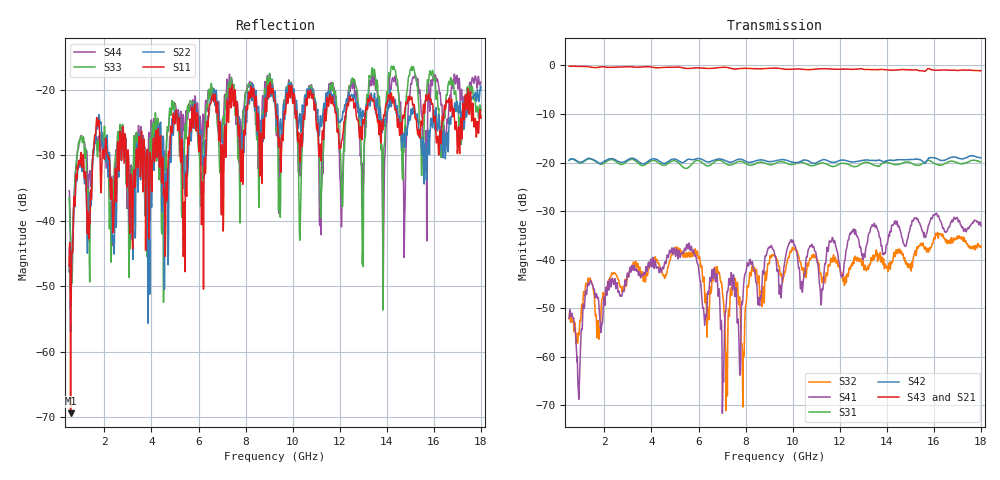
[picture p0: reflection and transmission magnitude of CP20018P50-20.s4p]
! Amtery
! Email: info@amtery.com
! Phone: 886-2-7730-0804
! Model Number: CP20018P-20
! 4-port S-parameter measurement data for Bi-Directional Coupler
! Frequency Range: 0.5 GHz to 18 GHz
! Port 1: Input
! Port 2: Output
! Port 3: Coupled Forward
! Port 4: Coupled Reverse
# hz S ma R 50
! freq  magS11  angS11  magS12  angS12  magS13  angS13  magS14  angS14
!  magS21  angS21  magS22  angS22  magS23  angS23  magS24  angS24
!  magS31  angS31  magS32  angS32  magS33  angS33  magS34  angS34
!  magS41  angS41  magS42  angS42  magS43  angS43  magS44  angS44
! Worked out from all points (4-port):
!   1401 points, 500 MHz to 18 GHz, reference 50 ohm
!   strongest paths, dB at 500 MHz, 4.875 GHz, 9.25 GHz, 13.62 GHz, 18 GHz:
!     S43: -0.1, -0.4, -0.5, -0.9, -1.1
!     S21: -0.1, -0.4, -0.7, -0.7, -1.0
!     S42: -19.5, -19.3, -19.7, -19.5, -19.0
!     S31: -19.5, -19.7, -20.2, -20.7, -19.8
!     S41: -52.1, -37.5, -39.4, -34.0, -33.0
!     S32: -52.1, -39.0, -39.2, -39.1, -37.1
!   lowest |S11| = -69.4 dB at 562.5 MHz (marker M1), VSWR 1.00, Z = 50 + j0.0339 ohm
!   |S11| at or under -10 dB: start of sweep to end of sweep
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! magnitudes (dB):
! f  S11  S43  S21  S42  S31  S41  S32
! 500 MHz  -46.9  -0.1  -0.1  -19.5  -19.5  -52.1  -52.1
! 562.5 MHz  -69.4  -0.2  -0.1  -19.3  -19.3  -51.2  -52.9
! 1.7 GHz  -25.0  -0.4  -0.5  -19.9  -20.0  -47.9  -54.8
! 3.925 GHz  -31.4  -0.3  -0.4  -19.5  -19.8  -41.5  -41.3
! 7.013 GHz  -28.4  -0.4  -0.5  -19.3  -19.7  -71.6  -46.4
! 9.037 GHz  -19.1  -0.6  -0.7  -19.8  -20.4  -37.5  -39.3
! 18 GHz  -24.0  -1.1  -1.0  -19.0  -19.8  -33.0  -37.1
